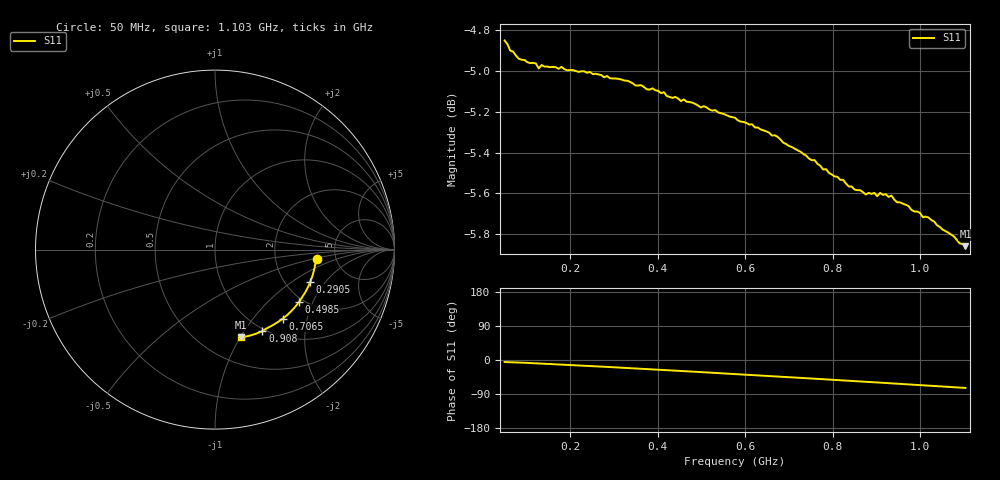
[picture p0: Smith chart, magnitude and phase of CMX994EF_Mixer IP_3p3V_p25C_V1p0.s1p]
! CMX994EF, Mixer Input s-parameters at Vcc = 3.3V, de-embedded to DUT
! Created: GMT 2025-07-21 08:55:05
# Hz S MA R 50
! freq[Hz]  S11[mag]  S11[ang]
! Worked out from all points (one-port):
!   163 points, 50 MHz to 1.103 GHz, reference 50 ohm
!   lowest |S11| = -5.9 dB at 1.103 GHz (marker M1), VSWR 3.08, Z = 38 - j50.2 ohm
!   |S11| at or under -10 dB: nowhere
!   S11 on the Smith chart (normalised r, x): 50 MHz: 3.58, -0.57; 290.5 MHz: 2.72, -1.42; 498.5 MHz: 1.89, -1.58; 706.5 MHz: 1.32, -1.44; 908 MHz: 0.97, -1.21; 1.103 GHz: 0.76, -1.00
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5e7  0.5722 -5.3
6.3e7  0.5689 -5.9
8.9e7  0.566 -6.9
1.215e8  0.5648 -8.6
1.28e8  0.5632 -9.0
1.345e8  0.5643 -9.4
1.865e8  0.563 -12.4
2.45e8  0.5621 -15.9
2.905e8  0.5601 -18.6
3.165e8  0.5597 -20.3
3.88e8  0.5569 -24.8
4.465e8  0.5537 -28.5
4.985e8  0.5509 -31.9
5.18e8  0.5503 -33.3
5.765e8  0.5477 -37.0
6.155e8  0.5457 -39.7
6.545e8  0.5431 -42.0
7.065e8  0.5387 -45.6
7.13e8  0.5382 -46.0
7.715e8  0.533 -50.0
8.105e8  0.5297 -53.0
8.43e8  0.5268 -55.3
9.015e8  0.5239 -59.2
9.08e8  0.5249 -59.7
9.73e8  0.521 -64.5
1.032e9  0.5164 -68.5
1.064e9  0.5132 -71.0
1.103e9  0.5093 -73.7
